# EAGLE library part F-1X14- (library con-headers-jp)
FEMALE HEADER
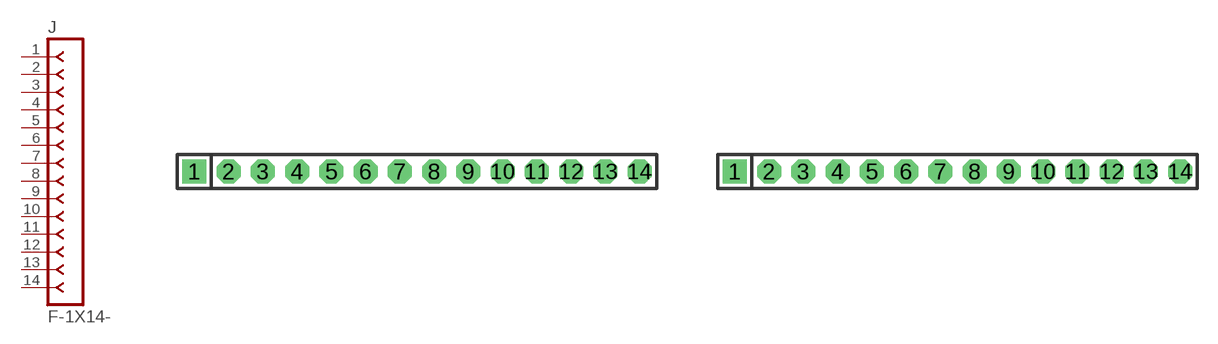
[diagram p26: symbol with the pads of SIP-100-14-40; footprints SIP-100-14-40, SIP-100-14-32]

Designator prefix J

## F-1X14-SIP-100-40  [SIP-100-14-40]
1  1  pas
2  2  pas
3  3  pas
4  4  pas
5  5  pas
6  6  pas
7  7  pas
8  8  pas
9  9  pas
10  10  pas
11  11  pas
12  12  pas
13  13  pas
14  14  pas

## F-1X14-SIP-100-32  [SIP-100-14-32]
Pads as for SIP-100-14-40

## F-1X14-SIP-100-32Y  [SIP-100-14-32Y]
Pads as for SIP-100-14-40

## F-1X14-SIP-100-40Y  [SIP-100-14-40Y]
Pads as for SIP-100-14-40

## F-1X14-KK-4455-B14  [KK-4455-B14]
Pads as for SIP-100-14-40

## F-1X14-KK-4455-C14  [KK-4455-C14]
Pads as for SIP-100-14-40

## F-1X14-KK-4455-A14  [KK-4455-A14]
Pads as for SIP-100-14-40

## Footprint SIP-100-14-40 (pad centres in mm)
SIP Header - 0.1", 40 mil drill
drill 1.016 pad 1.778 square: 1 -16.51,0
drill 1.016 pad 1.778 octagon: 2 -13.97,0; 3 -11.43,0; 4 -8.89,0; 5 -6.35,0; 6 -3.81,0; 7 -1.27,0; 8 1.27,0; 9 3.81,0; 10 6.35,0; 11 8.89,0; 12 11.43,0; 13 13.97,0; 14 16.51,0

## Footprint SIP-100-14-32 (pad centres in mm)
SIP Header - 0.1", 32 mil drill
drill 0.813 pad 1.778 square: 1 -16.51,0
drill 0.813 pad 1.778 octagon: 2 -13.97,0; 3 -11.43,0; 4 -8.89,0; 5 -6.35,0; 6 -3.81,0; 7 -1.27,0; 8 1.27,0; 9 3.81,0; 10 6.35,0; 11 8.89,0; 12 11.43,0; 13 13.97,0; 14 16.51,0

## Footprint SIP-100-14-32Y (pad centres in mm)
SIP Header - 0.1", 32 mil drill
drill 0.813 long: 1 -16.51,0; 2 -13.97,0; 3 -11.43,0; 4 -8.89,0; 5 -6.35,0; 6 -3.81,0; 7 -1.27,0; 8 1.27,0; 9 3.81,0; 10 6.35,0; 11 8.89,0; 12 11.43,0; 13 13.97,0; 14 16.51,0

## Footprint SIP-100-14-40Y (pad centres in mm)
SIP Header - 0.1", 40 mil drill
drill 1.016 long: 1 -16.51,0; 2 -13.97,0; 3 -11.43,0; 4 -8.89,0; 5 -6.35,0; 6 -3.81,0; 7 -1.27,0; 8 1.27,0; 9 3.81,0; 10 6.35,0; 11 8.89,0; 12 11.43,0; 13 13.97,0; 14 16.51,0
